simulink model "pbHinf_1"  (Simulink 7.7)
settings: Solver=ode45  StartTime=0.0  StopTime=10.0  RelTol=1e-3
libraries: cstblocks x2

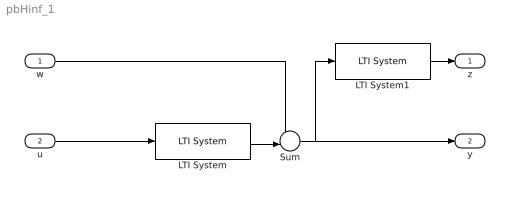
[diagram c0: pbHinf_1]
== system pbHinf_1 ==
  w : Inport
  u : Inport  Port=2
  LTI System : cstblocks/LTI System  SystemSampleTime=-1  sys=G  IC=[]
  LTI System1 : cstblocks/LTI System  SystemSampleTime=-1  sys=W1  IC=[]
  Sum : Sum  Inputs=+-|
  z : Outport
  y : Outport  Port=2
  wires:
  LTI System/1 -> Sum/2
  w/1 -> Sum/1
  u/1 -> LTI System/1
  LTI System1/1 -> z/1
  Sum/1 -> y/1, LTI System1/1
